| IBIS file stm32f413_f423_ufbga100.ibs
[IBIS ver] 4.2
[File name] stm32f413_f423_ufbga100.ibs
[File Rev] 1.2
[Date]  18-05-2020
[Source] Data Created at STMicroelectronics
[Notes]  File originated from ELDO simulations. rev 1.1: removal of the rising/falling waveform I2C
[Disclaimer]  This information is for modeling purpose only and is
   not guaranted. The information is subject to change without
   notice.
[Copyright] Copyright 2020 STMicroelectronics Inc.
|   Component stm32f413_f423_ufbga100
[Component] stm32f413_f423_ufbga100
[Manufacturer] STMicroelectronics
[Package]
| variable   typ   min   max
R_pkg   0.0   0.0   0.0
L_pkg   0.0H   0.0H   0.0H
C_pkg   0.0F   0.0F   0.0F
[Pin]  signal_name   model_name   R_pin   L_pin   C_pin
A1 PE3 io8usb_lsfs_otg_ft
A10 PA14 io8p_arsudq_ft
A11 PA13 io8p_arsudq_ft
A12 PA12 io8usb_lsfs_otg_ft
A2 PE1 io8p_arsudq_ft
A3 PB8 io8p_arsudq_i2cin_ft
A4 BOOT0 vpp_test_hv
A5 PD7 io8p_arsudq_ft
A6 PD5 io8p_arsudq_ft
A7 PB4 io8p_arsudq_i2cin_ft
A8 PB3 io8p_arsudq_i2c_ft
A9 PA15 io8p_arsudq_ft
B1 PE4 io8p_arsudq_ft
B10 PC12 io8p_arsudq_ft
B11 PC10 io8p_arsudq_ft
B12 PA11 io8usb_lsfs_otg_ft
B2 PE2 io8p_arsudq_ft
B3 PB9 io8p_arsudq_i2cin_ft
B4 PB7 io8p_arsudq_i2cin_ft
B5 PB6 io8p_arsudq_i2cin_ft
B6 PD6 io8p_arsudq_ft
B7 PD4 io8p_arsudq_ft
B8 PD3 io8p_arsudq_ft
B9 PD1 io8p_arsudq_ft
C1 PC13-ANTI_TAMP io8p_arwsudq_ft_v33
C10 PC11 io8p_arsudq_ft
C11 VCAP2_0 POWER
C12 PA10 io8usb_id_otg_ft
C2 PE5 io8p_arsudq_ft
C3 PE0 io8p_arsudq_ft
C4 VDD_3 POWER
C5 PB5 io8p_ar3wsudq_ft
C8 PD2 io8p_arsudq_ft
C9 PD0 io8p_arsudq_ft
D1 PC14-OSC32_IN io8p_arwsudq_ft
D10 PA9 io8usb_vbus_otg_ft
D11 PA8 io8p_arsudq_i2cin_ft
D12 PC9 io8p_arsudq_i2cin_ft
D2 PE6 io8p_arsudq_ft
D3 VSS_3 GND
E1 PC15-OSC32_OUT io8p_arsudq_ft
E10 PC8 io8p_arsudq_ft
E11 PC7 io8p_arsudq_i2c_ft
E12 PC6 io8p_arsudq_i2c_ft
E2 VBAT POWER
E3 BYPASS_USER GND
F1 PH0-OSC_IN io8p_arsudq_ft
F11 VSS_2_0 GND
F12 VSS_1_0 GND
F2 VSS_5 GND
G1 PH1-OSC_OUT io8p_arsudq_ft
G11 VDD_SA_2 POWER
G12 VDD_1_0 POWER
G2 VDD_5 POWER
H1 PC0 io8p_arwsudq_ft_v33
H10 PD15 io8p_arsudq_i2c_ft
H11 PD14 io8p_arsudq_i2c_ft
H12 PD13 io8p_arsudq_i2c_ft
H2 NRST ioreset_ft_v33
H3 PDR_ON GND
J1 VSSA GND
J10 PD12 io8p_arsudq_i2c_ft
J11 PD11 io8p_arsudq_ft
J12 PD10 io8p_arsudq_ft
J2 PC1 io8p_arwsudq_ft_v33
J3 PC2 io8p_arwsudq_ft
K1 VREF- GND
K10 PB15 io8p_arsudq_i2c_ft
K11 PB14 io8p_arsudq_i2c_ft
K12 PB13 io8p_arsudq_ft
K2 PC3 io8p_arwsudq_ft
K3 PA2 io8p_arwsudq_ft
K4 PA5 io8p_ar3wsudq_ft
K5 PC4 io8p_arwsudq_ft
K8 PD9 io8p_arsudq_ft
K9 PB11 io8p_arsudq_i2cin_ft
L1 VREF+ POWER
L10 PB10 io8p_arsudq_i2c_ft
L11 VCAP1_0 POWER
L12 PB12 io8p_arsudq_ft
L2 PA0-WKUP io8p_arwsudq_ft_v33
L3 PA3 io8p_arwsudq_ft
L4 PA6 io8p_ar3wsudq_ft
L5 PC5 io8p_arwsudq_ft
L6 PB2 io8p_arwsudq_ft
L7 PE8 io8p_arsudq_ft
L8 PE10 io8p_arsudq_ft
L9 PE12 io8p_arsudq_ft
M1 VDDA POWER
M10 PE13 io8p_arsudq_ft
M11 PE14 io8p_arsudq_ft
M12 PE15 io8p_ar3wsudq_ft
M2 PA1 io8p_arwsudq_ft
M3 PA4 io8p_ar3wsudq_ft
M4 PA7 io8p_arwsudq_ft
M5 PB0 io8p_ar3wsudq_ft
M6 PB1 io8p_ar3wsudq_ft
M7 PE7 io8p_arsudq_ft
M8 PE9 io8p_arsudq_ft
M9 PE11 io8p_arsudq_ft
[Model Selector] io8p_ar3wsudq_ft
io8p00_ar3wsudq_ft_pd_lv  "SPEED00 1P8V, PD=40kOhm"
io8p00_ar3wsudq_ft_pu_lv  "SPEED00 1P8V, PU=40kOhm"
io8p00_ar3wsudq_ft_lv  "SPEED00 1P8V"
io8p01_ar3wsudq_ft_pd_lv  "SPEED01 1P8V, PD=40kOhm"
io8p01_ar3wsudq_ft_pu_lv  "SPEED01 1P8V, PU=40kOhm"
io8p01_ar3wsudq_ft_lv  "SPEED01 1P8V"
io8p10_ar3wsudq_ft_pd_lv  "SPEED10 1P8V, PD=40kOhm"
io8p10_ar3wsudq_ft_pu_lv  "SPEED10 1P8V, PU=40kOhm"
io8p10_ar3wsudq_ft_lv  "SPEED10 1P8V"
io8p11_ar3wsudq_ft_pd_lv  "SPEED11 1P8V, PD=40kOhm"
io8p11_ar3wsudq_ft_pu_lv  "SPEED11 1P8V, PU=40kOhm"
io8p11_ar3wsudq_ft_lv  "SPEED11 1P8V"
io8p00_ar3wsudq_ft_pd  "SPEED00, PD=40kOhm"
io8p00_ar3wsudq_ft_pu  "SPEED00, PU=40kOhm"
io8p00_ar3wsudq_ft  "SPEED00"
io8p01_ar3wsudq_ft_pd  "SPEED01, PD=40kOhm"
io8p01_ar3wsudq_ft_pu  "SPEED01, PU=40kOhm"
io8p01_ar3wsudq_ft  "SPEED01"
io8p10_ar3wsudq_ft_pd  "SPEED10, PD=40kOhm"
io8p10_ar3wsudq_ft_pu  "SPEED10, PU=40kOhm"
io8p10_ar3wsudq_ft  "SPEED10"
io8p11_ar3wsudq_ft_pd  "SPEED11, PD=40kOhm"
io8p11_ar3wsudq_ft_pu  "SPEED11, PU=40kOhm"
io8p11_ar3wsudq_ft  "SPEED11"
[Model Selector] io8p_arsudq_ft
io8p00_arsudq_ft_pd_lv  "SPEED00 1P8V, PD=40kOhm"
io8p00_arsudq_ft_pu_lv  "SPEED00 1P8V, PU=40kOhm"
io8p00_arsudq_ft_lv  "SPEED00 1P8V"
io8p01_arsudq_ft_pd_lv  "SPEED01 1P8V, PD=40kOhm"
io8p01_arsudq_ft_pu_lv  "SPEED01 1P8V, PU=40kOhm"
io8p01_arsudq_ft_lv  "SPEED01 1P8V"
io8p10_arsudq_ft_pd_lv  "SPEED10 1P8V, PD=40kOhm"
io8p10_arsudq_ft_pu_lv  "SPEED10 1P8V, PU=40kOhm"
io8p10_arsudq_ft_lv  "SPEED10 1P8V"
io8p11_arsudq_ft_pd_lv  "SPEED11 1P8V, PD=40kOhm"
io8p11_arsudq_ft_pu_lv  "SPEED11 1P8V, PU=40kOhm"
io8p11_arsudq_ft_lv  "SPEED11 1P8V"
io8p00_arsudq_ft_pd  "SPEED00, PD=40kOhm"
io8p00_arsudq_ft_pu  "SPEED00, PU=40kOhm"
io8p00_arsudq_ft  "SPEED00"
io8p01_arsudq_ft_pd  "SPEED01, PD=40kOhm"
io8p01_arsudq_ft_pu  "SPEED01, PU=40kOhm"
io8p01_arsudq_ft  "SPEED01"
io8p10_arsudq_ft_pd  "SPEED10, PD=40kOhm"
io8p10_arsudq_ft_pu  "SPEED10, PU=40kOhm"
io8p10_arsudq_ft  "SPEED10"
io8p11_arsudq_ft_pd  "SPEED11, PD=40kOhm"
io8p11_arsudq_ft_pu  "SPEED11, PU=40kOhm"
io8p11_arsudq_ft  "SPEED11"
[Model Selector] io8p_arsudq_i2c_ft
io8prog_1v8_i2c_pd  "5V Tol GPIO 1.8V range i2c functionality with pull down"
io8prog_1v8_i2c_pu  "5V Tol GPIO 1.8V range i2c functionality with pull up"
io8prog_1v8_i2c  "5V Tol GPIO 1.8V range i2c functionality"
io8prog_3v3_i2c_pd  "5V Tol GPIO 3.3V range i2c functionality with pull down"
io8prog_3v3_i2c_pu  "5V Tol GPIO 3.3V range i2c functionality with pull up"
io8prog_3v3_i2c  "5V Tol GPIO 3.3V range i2c functionality"
io8prog_1v8_pd_00  "5V Tol GPIO 1.8V range with pd speed 00"
io8prog_1v8_pu_00  "5V Tol GPIO 1.8V range with pu speed 00"
io8prog_1v8_00  "5V Tol GPIO 1.8V range speed 00"
io8prog_3v3_pd_00  "5V Tol GPIO 3.3V range with pd speed 00"
io8prog_3v3_pu_00  "5V Tol GPIO 3.3V range with pu speed 00"
io8prog_3v3_00  "5V Tol GPIO 3.3V range speed 00"
io8prog_1v8_pd_01  "5V Tol GPIO 1.8V range with pd speed 01"
io8prog_1v8_pu_01  "5V Tol GPIO 1.8V range with pu speed 01"
io8prog_1v8_01  "5V Tol GPIO 1.8V range speed 01"
io8prog_3v3_pd_01  "5V Tol GPIO 3.3V range with pd speed 01"
io8prog_3v3_pu_01  "5V Tol GPIO 3.3V range with pu speed 01"
io8prog_3v3_01  "5V Tol GPIO 3.3V range speed 01"
io8prog_1v8_pd_10  "5V Tol GPIO 1.8V range with pd speed 10"
io8prog_1v8_pu_10  "5V Tol GPIO 1.8V range with pu speed 10"
io8prog_1v8_10  "5V Tol GPIO 1.8V range speed 10"
io8prog_3v3_pd_10  "5V Tol GPIO 3.3V range with pd speed 10"
io8prog_3v3_pu_10  "5V Tol GPIO 3.3V range with pu speed 10"
io8prog_3v3_10  "5V Tol GPIO 3.3V range speed 10"
io8prog_1v8_pd_11  "5V Tol GPIO 1.8V range with pd speed 11"
io8prog_1v8_pu_11  "5V Tol GPIO 1.8V range with pu speed 11"
io8prog_1v8_11  "5V Tol GPIO 1.8V range speed 11"
io8prog_3v3_pd_11  "5V Tol GPIO 3.3V range with pd speed 11"
io8prog_3v3_pu_11  "5V Tol GPIO 3.3V range with pu speed 11"
io8prog_3v3_11  "5V Tol GPIO 3.3V range speed 11"
[Model Selector] io8p_arsudq_i2cin_ft
io8p00_arsudq_i2cin_ft_pd_lv  "SPEED00 1P8V, PD=40kOhm"
io8p00_arsudq_i2cin_ft_pu_lv  "SPEED00 1P8V, PU=40kOhm"
io8p00_arsudq_i2cin_ft_lv  "SPEED00 1P8V"
io8p01_arsudq_i2cin_ft_pd_lv  "SPEED01 1P8V, PD=40kOhm"
io8p01_arsudq_i2cin_ft_pu_lv  "SPEED01 1P8V, PU=40kOhm"
io8p01_arsudq_i2cin_ft_lv  "SPEED01 1P8V"
io8p10_arsudq_i2cin_ft_pd_lv  "SPEED10 1P8V, PD=40kOhm"
io8p10_arsudq_i2cin_ft_pu_lv  "SPEED10 1P8V, PU=40kOhm"
io8p10_arsudq_i2cin_ft_lv  "SPEED10 1P8V"
io8p11_arsudq_i2cin_ft_pd_lv  "SPEED11 1P8V, PD=40kOhm"
io8p11_arsudq_i2cin_ft_pu_lv  "SPEED11 1P8V, PU=40kOhm"
io8p11_arsudq_i2cin_ft_lv  "SPEED11 1P8V"
io8p00_arsudq_i2cin_ft_pd  "SPEED00, PD=40kOhm"
io8p00_arsudq_i2cin_ft_pu  "SPEED00, PU=40kOhm"
io8p00_arsudq_i2cin_ft  "SPEED00"
io8p01_arsudq_i2cin_ft_pd  "SPEED01, PD=40kOhm"
io8p01_arsudq_i2cin_ft_pu  "SPEED01, PU=40kOhm"
io8p01_arsudq_i2cin_ft  "SPEED01"
io8p10_arsudq_i2cin_ft_pd  "SPEED10, PD=40kOhm"
io8p10_arsudq_i2cin_ft_pu  "SPEED10, PU=40kOhm"
io8p10_arsudq_i2cin_ft  "SPEED10"
io8p11_arsudq_i2cin_ft_pd  "SPEED11, PD=40kOhm"
io8p11_arsudq_i2cin_ft_pu  "SPEED11, PU=40kOhm"
io8p11_arsudq_i2cin_ft  "SPEED11"
[Model Selector] io8p_arwsudq_ft
io8p00_arwsudq_ft_pd_lv  "SPEED00 1P8V, PD=40kOhm"
io8p00_arwsudq_ft_pu_lv  "SPEED00 1P8V, PU=40kOhm"
io8p00_arwsudq_ft_lv  "SPEED00 1P8V"
io8p01_arwsudq_ft_pd_lv  "SPEED01 1P8V, PD=40kOhm"
io8p01_arwsudq_ft_pu_lv  "SPEED01 1P8V, PU=40kOhm"
io8p01_arwsudq_ft_lv  "SPEED01 1P8V"
io8p10_arwsudq_ft_pd_lv  "SPEED10 1P8V, PD=40kOhm"
io8p10_arwsudq_ft_pu_lv  "SPEED10 1P8V, PU=40kOhm"
io8p10_arwsudq_ft_lv  "SPEED10 1P8V"
io8p11_arwsudq_ft_pd_lv  "SPEED11 1P8V, PD=40kOhm"
io8p11_arwsudq_ft_pu_lv  "SPEED11 1P8V, PU=40kOhm"
io8p11_arwsudq_ft_lv  "SPEED11 1P8V"
io8p00_arwsudq_ft_pd  "SPEED00, PD=40kOhm"
io8p00_arwsudq_ft_pu  "SPEED00, PU=40kOhm"
io8p00_arwsudq_ft  "SPEED00"
io8p01_arwsudq_ft_pd  "SPEED01, PD=40kOhm"
io8p01_arwsudq_ft_pu  "SPEED01, PU=40kOhm"
io8p01_arwsudq_ft  "SPEED01"
io8p10_arwsudq_ft_pd  "SPEED10, PD=40kOhm"
io8p10_arwsudq_ft_pu  "SPEED10, PU=40kOhm"
io8p10_arwsudq_ft  "SPEED10"
io8p11_arwsudq_ft_pd  "SPEED11, PD=40kOhm"
io8p11_arwsudq_ft_pu  "SPEED11, PU=40kOhm"
io8p11_arwsudq_ft  "SPEED11"
[Model Selector] io8p_arwsudq_ft_v33
io8p00_arwsudq_ft_v33_pd_lv  "SPEED00 1P8V, PD=40kOhm"
io8p00_arwsudq_ft_v33_pu_lv  "SPEED00 1P8V, PU=40kOhm"
io8p00_arwsudq_ft_v33_lv  "SPEED00 1P8V"
io8p01_arwsudq_ft_v33_pd_lv  "SPEED01 1P8V, PD=40kOhm"
io8p01_arwsudq_ft_v33_pu_lv  "SPEED01 1P8V, PU=40kOhm"
io8p01_arwsudq_ft_v33_lv  "SPEED01 1P8V"
io8p10_arwsudq_ft_v33_pd_lv  "SPEED10 1P8V, PD=40kOhm"
io8p10_arwsudq_ft_v33_pu_lv  "SPEED10 1P8V, PU=40kOhm"
io8p10_arwsudq_ft_v33_lv  "SPEED10 1P8V"
io8p11_arwsudq_ft_v33_pd_lv  "SPEED11 1P8V, PD=40kOhm"
io8p11_arwsudq_ft_v33_pu_lv  "SPEED11 1P8V, PU=40kOhm"
io8p11_arwsudq_ft_v33_lv  "SPEED11 1P8V"
io8p00_arwsudq_ft_v33_pd  "SPEED00, PD=40kOhm"
io8p00_arwsudq_ft_v33_pu  "SPEED00, PU=40kOhm"
io8p00_arwsudq_ft_v33  "SPEED00"
io8p01_arwsudq_ft_v33_pd  "SPEED01, PD=40kOhm"
io8p01_arwsudq_ft_v33_pu  "SPEED01, PU=40kOhm"
io8p01_arwsudq_ft_v33  "SPEED01"
io8p10_arwsudq_ft_v33_pd  "SPEED10, PD=40kOhm"
io8p10_arwsudq_ft_v33_pu  "SPEED10, PU=40kOhm"
io8p10_arwsudq_ft_v33  "SPEED10"
io8p11_arwsudq_ft_v33_pd  "SPEED11, PD=40kOhm"
io8p11_arwsudq_ft_v33_pu  "SPEED11, PU=40kOhm"
io8p11_arwsudq_ft_v33  "SPEED11"
[Model Selector] io8usb_id_otg_ft
io8p00_id_otg_ft_pd_lv  "SPEED00 1P8V, PD=14kOhm"
io8p00_id_otg_ft_pu_lv  "SPEED00 1P8V, PU=14kOhm"
io8p00_id_otg_ft_lv  "SPEED00 1P8V"
io8p01_id_otg_ft_pd_lv  "SPEED01 1P8V, PD=14kOhm"
io8p01_id_otg_ft_pu_lv  "SPEED01 1P8V, PU=14kOhm"
io8p01_id_otg_ft_lv  "SPEED01 1P8V"
io8p10_id_otg_ft_pd_lv  "SPEED10 1P8V, PD=14kOhm"
io8p10_id_otg_ft_pu_lv  "SPEED10 1P8V, PU=14kOhm"
io8p10_id_otg_ft_lv  "SPEED10 1P8V"
io8p11_id_otg_ft_pd_lv  "SPEED11 1P8V, PD=14kOhm"
io8p11_id_otg_ft_pu_lv  "SPEED11 1P8V, PU=14kOhm"
io8p11_id_otg_ft_lv  "SPEED11 1P8V"
io8p00_id_otg_ft_pd  "SPEED00, PD=14kOhm"
io8p00_id_otg_ft_pu  "SPEED00, PU=14kOhm"
io8p00_id_otg_ft  "SPEED00"
io8p01_id_otg_ft_pd  "SPEED01, PD=14kOhm"
io8p01_id_otg_ft_pu  "SPEED01, PU=14kOhm"
io8p01_id_otg_ft  "SPEED01"
io8p10_id_otg_ft_pd  "SPEED10, PD=14kOhm"
io8p10_id_otg_ft_pu  "SPEED10, PU=14kOhm"
io8p10_id_otg_ft  "SPEED10"
io8p11_id_otg_ft_pd  "SPEED11, PD=14kOhm"
io8p11_id_otg_ft_pu  "SPEED11, PU=14kOhm"
io8p11_id_otg_ft  "SPEED11"
[Model Selector] io8usb_lsfs_otg_ft
io8usb_ls_otg_ft_dpdn_pd  "LS USB DP/DN IO + PD=20kOhm"
io8usb_ls_otg_ft_dpdn_pupu2  "LS USB DP/DN IO + PU/PU2=2.2kOhm"
io8usb_ls_otg_ft_dpdn_pu2  "LS USB DP/DN IO + PU2=1.2kOhm"
io8usb_ls_otg_ft_dpdn_pu  "LS USB DP/DN IO + PU=1.2kOhm"
io8usb_ls_otg_ft_dpdn  "LS USB DP/DN IO"
io8usb_fs_otg_ft_dpdn_pd  "HS USB DP/DN IO + PD=20kOhm"
io8usb_fs_otg_ft_dpdn_pupu2  "HS USB DP/DN IO + PU/PU2=2.2kOhm"
io8usb_fs_otg_ft_dpdn_pu2  "HS USB DP/DN IO + PU2=1.2kOhm"
io8usb_fs_otg_ft_dpdn_pu  "HS USB DP/DN IO + PU=1.2kOhm"
io8usb_fs_otg_ft_dpdn  "HS USB DP/DN IO"
io8p00_lsfs_otg_ft_pd_lv  "SPEED00 1P8V, PD=40kOhm"
io8p00_lsfs_otg_ft_pu_lv  "SPEED00 1P8V, PU=40kOhm"
io8p00_lsfs_otg_ft_lv  "SPEED00 1P8V"
io8p01_lsfs_otg_ft_pd_lv  "SPEED01 1P8V, PD=40kOhm"
io8p01_lsfs_otg_ft_pu_lv  "SPEED01 1P8V, PU=40kOhm"
io8p01_lsfs_otg_ft_lv  "SPEED01 1P8V"
io8p10_lsfs_otg_ft_pd_lv  "SPEED10 1P8V, PD=40kOhm"
io8p10_lsfs_otg_ft_pu_lv  "SPEED10 1P8V, PU=40kOhm"
io8p10_lsfs_otg_ft_lv  "SPEED10 1P8V"
io8p11_lsfs_otg_ft_pd_lv  "SPEED11 1P8V, PD=40kOhm"
io8p11_lsfs_otg_ft_pu_lv  "SPEED11 1P8V, PU=40kOhm"
io8p11_lsfs_otg_ft_lv  "SPEED11 1P8V"
io8p00_lsfs_otg_ft_pd  "SPEED00, PD=40kOhm"
io8p00_lsfs_otg_ft_pu  "SPEED00, PU=40kOhm"
io8p00_lsfs_otg_ft  "SPEED00"
io8p01_lsfs_otg_ft_pd  "SPEED01, PD=40kOhm"
io8p01_lsfs_otg_ft_pu  "SPEED01, PU=40kOhm"
io8p01_lsfs_otg_ft  "SPEED01"
io8p10_lsfs_otg_ft_pd  "SPEED10, PD=40kOhm"
io8p10_lsfs_otg_ft_pu  "SPEED10, PU=40kOhm"
io8p10_lsfs_otg_ft  "SPEED10"
io8p11_lsfs_otg_ft_pd  "SPEED11, PD=40kOhm"
io8p11_lsfs_otg_ft_pu  "SPEED11, PU=40kOhm"
io8p11_lsfs_otg_ft  "SPEED11"
[Model Selector] io8usb_vbus_otg_ft
io8psenb_vbus_otg_ft  "VBUS PULSE, SENSE VB"
io8psenab_vbus_otg_ft  "VBUS PULSE, SENSE VA and VB"
io8psena_vbus_otg_ft  "VBUS PULSE, SENSE VA"
io8psen_vbus_otg_ft  "VBUS PULSE"
io8p00_vbus_otg_ft_pd_lv  "SPEED00 1P8V, PD=40kOhm"
io8p00_vbus_otg_ft_pu_lv  "SPEED00 1P8V, PU=40kOhm"
io8p00_vbus_otg_ft_lv  "SPEED00 1P8V"
io8p01_vbus_otg_ft_pd_lv  "SPEED01 1P8V, PD=40kOhm"
io8p01_vbus_otg_ft_pu_lv  "SPEED01 1P8V, PU=40kOhm"
io8p01_vbus_otg_ft_lv  "SPEED01 1P8V"
io8p10_vbus_otg_ft_pd_lv  "SPEED10 1P8V, PD=40kOhm"
io8p10_vbus_otg_ft_pu_lv  "SPEED10 1P8V, PU=40kOhm"
io8p10_vbus_otg_ft_lv  "SPEED10 1P8V"
io8p11_vbus_otg_ft_pd_lv  "SPEED11 1P8V, PD=40kOhm"
io8p11_vbus_otg_ft_pu_lv  "SPEED11 1P8V, PU=40kOhm"
io8p11_vbus_otg_ft_lv  "SPEED11 1P8V"
io8p00_vbus_otg_ft_pd  "SPEED00, PD=40kOhm"
io8p00_vbus_otg_ft_pu  "SPEED00, PU=40kOhm"
io8p00_vbus_otg_ft  "SPEED00"
io8p01_vbus_otg_ft_pd  "SPEED01, PD=40kOhm"
io8p01_vbus_otg_ft_pu  "SPEED01, PU=40kOhm"
io8p01_vbus_otg_ft  "SPEED01"
io8p10_vbus_otg_ft_pd  "SPEED10, PD=40kOhm"
io8p10_vbus_otg_ft_pu  "SPEED10, PU=40kOhm"
io8p10_vbus_otg_ft  "SPEED10"
io8p11_vbus_otg_ft_pd  "SPEED11, PD=40kOhm"
io8p11_vbus_otg_ft_pu  "SPEED11, PU=40kOhm"
io8p11_vbus_otg_ft  "SPEED11"
[Model Selector] ioreset_ft_v33
ioreset_ft_v33_pu_lv  "IORESET 1P8V + PU=40kOhm"
ioreset_ft_v33_nopu_lv  "IORESET 1P8V"
ioreset_ft_v33_pu  "IORESET + PU=40kOhm"
ioreset_ft_v33_nopu  "IORESET"
[Model Selector] vpp_test_hv
vpp_test_hv_2p4  "Input Buffer 1P8V"
vpp_test_hv_3p3  "Input Buffer"
| Models and submodels in the file (242): io8p00_ar3wsudq_ft_pd_lv (I/O), io8p00_ar3wsudq_ft_pu_lv (I/O), io8p00_ar3wsudq_ft_lv (I/O), io8p01_ar3wsudq_ft_pd_lv (I/O), io8p01_ar3wsudq_ft_pu_lv (I/O), io8p01_ar3wsudq_ft_lv (I/O), io8p10_ar3wsudq_ft_pd_lv (I/O), io8p10_ar3wsudq_ft_pu_lv (I/O), io8p10_ar3wsudq_ft_lv (I/O), io8p11_ar3wsudq_ft_pd_lv (I/O), io8p11_ar3wsudq_ft_pu_lv (I/O), io8p11_ar3wsudq_ft_lv (I/O), io8p00_ar3wsudq_ft_pd (I/O), io8p00_ar3wsudq_ft_pu (I/O), io8p00_ar3wsudq_ft (I/O), io8p01_ar3wsudq_ft_pd (I/O), io8p01_ar3wsudq_ft_pu (I/O), io8p01_ar3wsudq_ft (I/O), io8p10_ar3wsudq_ft_pd (I/O), io8p10_ar3wsudq_ft_pu (I/O), io8p10_ar3wsudq_ft (I/O), io8p11_ar3wsudq_ft_pd (I/O), io8p11_ar3wsudq_ft_pu (I/O), io8p11_ar3wsudq_ft (I/O), io8p00_arsudq_ft_pd_lv (I/O), io8p00_arsudq_ft_pu_lv (I/O), io8p00_arsudq_ft_lv (I/O), io8p01_arsudq_ft_pd_lv (I/O), io8p01_arsudq_ft_pu_lv (I/O), io8p01_arsudq_ft_lv (I/O), io8p10_arsudq_ft_pd_lv (I/O), io8p10_arsudq_ft_pu_lv (I/O), io8p10_arsudq_ft_lv (I/O), io8p11_arsudq_ft_pd_lv (I/O), io8p11_arsudq_ft_pu_lv (I/O), io8p11_arsudq_ft_lv (I/O), io8p00_arsudq_ft_pd (I/O), io8p00_arsudq_ft_pu (I/O), io8p00_arsudq_ft (I/O), io8p01_arsudq_ft_pd (I/O), io8p01_arsudq_ft_pu (I/O), io8p01_arsudq_ft (I/O), io8p10_arsudq_ft_pd (I/O), io8p10_arsudq_ft_pu (I/O), io8p10_arsudq_ft (I/O), io8p11_arsudq_ft_pd (I/O), io8p11_arsudq_ft_pu (I/O), io8p11_arsudq_ft (I/O), io8prog_1v8_i2c_pd (I/O), io8prog_1v8_i2c_pu (I/O), io8prog_1v8_i2c (I/O), io8prog_3v3_i2c_pd (I/O), io8prog_3v3_i2c_pu (I/O), io8prog_3v3_i2c (I/O), io8prog_1v8_pd_00 (I/O), io8prog_1v8_pu_00 (I/O), io8prog_1v8_00 (I/O), io8prog_3v3_pd_00 (I/O), io8prog_3v3_pu_00 (I/O), io8prog_3v3_00 (I/O), io8prog_1v8_pd_01 (I/O), io8prog_1v8_pu_01 (I/O), io8prog_1v8_01 (I/O), io8prog_3v3_pd_01 (I/O), io8prog_3v3_pu_01 (I/O), io8prog_3v3_01 (I/O), io8prog_1v8_pd_10 (I/O), io8prog_1v8_pu_10 (I/O), io8prog_1v8_10 (I/O), io8prog_3v3_pd_10 (I/O), io8prog_3v3_pu_10 (I/O), io8prog_3v3_10 (I/O), io8prog_1v8_pd_11 (I/O), io8prog_1v8_pu_11 (I/O), io8prog_1v8_11 (I/O), io8prog_3v3_pd_11 (I/O), io8prog_3v3_pu_11 (I/O), io8prog_3v3_11 (I/O), io8p00_arsudq_i2cin_ft_pd_lv (I/O), io8p00_arsudq_i2cin_ft_pu_lv (I/O)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
